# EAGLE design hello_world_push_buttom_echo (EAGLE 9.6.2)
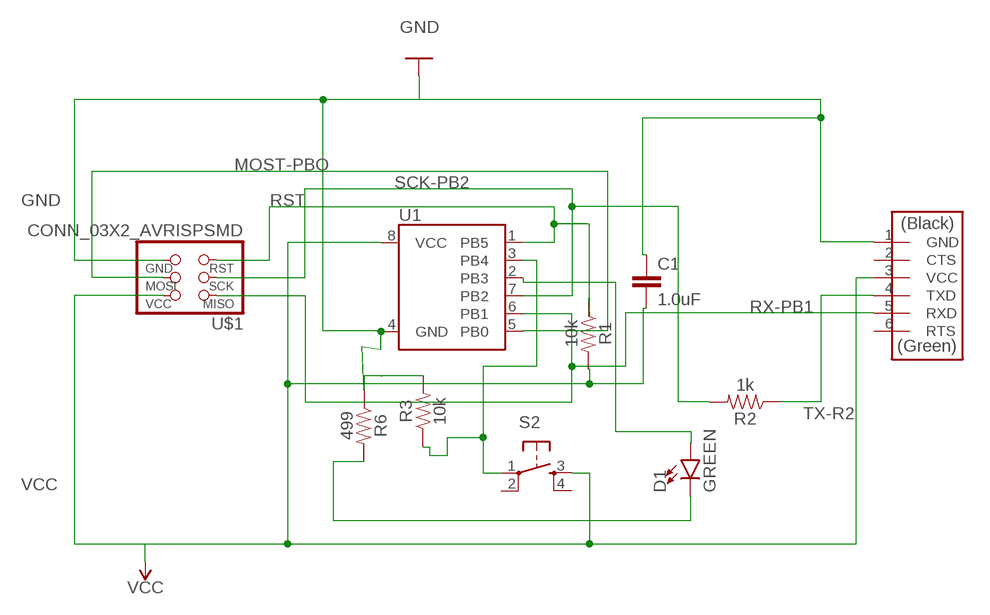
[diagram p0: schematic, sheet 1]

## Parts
C1  1.0uF  1.0UF-1206-50V-10%  [1206]
D1  GREEN  LED-GREEN1206  [LED-1206]
R1  10k  10OHM-1206-1/4W-1%  [1206]
R2  1k  10OHM-1206-1/4W-1%  [1206]
R3  10k  10OHM-1206-1/4W-1%  [1206]
R6  499  10OHM-1206-1/4W-1%  [1206]
S2  6MM_SWITCH6MM_SWITCH  [6MM_SWITCH]
U1  ATTINY85  [ATTINY85]
U$1  CONN_03X2_AVRISPSMD  [2X03SMD]
U$2  CONN_06_FTDI-SMD-HEADER  [1X06SMD]

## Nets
GND: C1.1 R3.2 R6.1 U1.4(GND) U$1.6(GND) U$2.1(GND)
MOST-PBO: U1.5(PB0) U$1.4(MOSI)
N$3: R3.1 S2.1(P) U1.3(PB4)
N$10: D1.A U1.2(PB3)
N$11: D1.C R6.2
RST: R1.1 U1.1(PB5) U$1.5(RST)
RX-PB1: U1.6(PB1) U$1.1(MISO) U$2.5(RXD)
SCK-PB2: R2.2 U1.7(PB2) U$1.3(SCK)
TX-R2: R2.1 U$2.4(TXD)
VCC: C1.2 R1.2 S2.3(S) U1.8(VCC) U$1.2(VCC) U$2.3(VCC)
Unconnected: S2.2(P1) S2.4(S1) U$2.2(CTS) U$2.6(RTS)

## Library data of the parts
C1 = SparkFun-Capacitors:1.0UF: 1µF ceramic capacitors; PROD_ID: CAP-09822
D1 = SparkFun-LED:LED-GREEN: Green SMD LED; PROD_ID: DIO-00862
R1-R3 R6 = SparkFun-Resistors:10OHM: 10Ω resistor; PROD_ID: RES-08705; VALUE: 10
S2 = fab:6MM_SWITCH: OMRON SWITCH
U1 = SparkFun-IC-Microcontroller:ATTINY85; PROD_ID: IC-09092
U$1 = fab:CONN_03X2_AVRISP
U$2 = fab:CONN_06_FTDI-SMD-HEADER

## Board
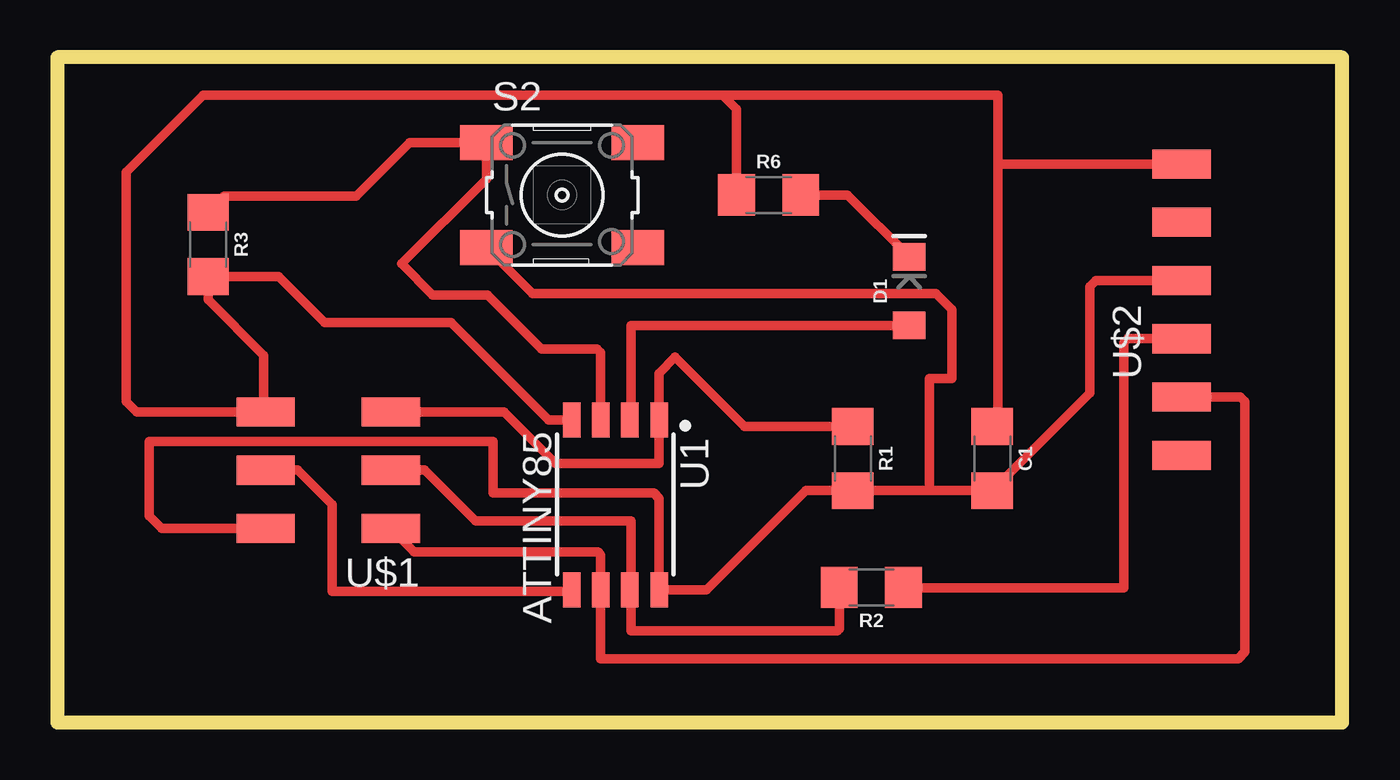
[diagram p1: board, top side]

Size 56 x 29 mm. Coordinates in mm from the lower left corner, seen from the top.
Outline: 0,0 56,0 56,29 0,29 0,0
Copper layers (1*16): Top 0.035mm / dielectric 1.5mm / Bottom 0.035mm
Design rules "default": minimum track width 6mil, minimum drill 0.35mm, track to track 6mil, track to pad 6mil, pad to pad 6mil, via to via 6mil, smd to smd 6mil, copper to edge 40mil, drill to drill 6mil, minimum pad ring 10mil, minimum via ring 8mil, stop-mask expansion 4mil, vias tented up to drill 0mil, thermal gap 10mil

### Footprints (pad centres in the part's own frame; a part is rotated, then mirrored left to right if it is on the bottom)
1206 = smd 1.6 x 1.8: 1 -1.4,0; 2 1.4,0
LED-1206 = smd 1.2 x 1.4: A -1.5,0; C 1.5,0
6MM_SWITCH = smd 2.286 x 1.524: 1 -3.302,2.286; 2 3.302,2.286; 3 -3.302,-2.286; 4 3.302,-2.286
ATTINY85 = smd 1.524 x 0.762: 1 -3.683,1.905; 2 -3.683,0.635; 3 -3.683,-0.635; 4 -3.683,-1.905; 5 3.727,-1.905; 6 3.727,-0.635; 7 3.727,0.635; 8 3.727,1.905
2X03SMD = smd 2.54 x 1.27: 1 -2.54,2.54; 2 2.92,2.54; 3 -2.54,0; 4 2.92,0; 5 -2.54,-2.54; 6 2.92,-2.54
1X06SMD = smd 2.54 x 1.27: 1 0,6.35; 2 0,3.81; 3 0,1.27; 4 0,-1.27; 5 0,-3.81; 6 0,-6.35

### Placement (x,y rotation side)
C1  40.75,11.51 270 top
D1  37.13,18.81 90 top
R1  34.67,11.51 270 top
R2  35.48,5.89 180 top
R3  6.57,20.84 270 top
R6  31,23 0 top
S2  22,23 0 top
U1  24.32,9.51 270 top
U$1  12,11 180 top
U$2  49,18 0 top

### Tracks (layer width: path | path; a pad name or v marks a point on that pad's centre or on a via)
GND
  Top 0.406: 29,27.35 6.35,27.35 3,24 3,14 3.46,13.54 U$1.6 9,13.62 9,16 6.57,18.43 R3.2 9.64,19.44 11.64,17.44 17.17,17.44 21.41,13.19 U1.4 | 29,27.35 41,27.35 41,24.35 | 41,24.35 U$2.1 | C1.1 41,13.16 41,24.35 | R6.1 29.6,26.75 29,27.35
MOST-PBO
  Top 0.406: U$1.4 10.48,11 11.98,9.5 11.98,5.71 22.34,5.71 U1.5
N$3
  Top 0.406: R3.1 7.28,22.95 13.01,22.95 15.35,25.29 S2.1 18.7,23.7 15,20 16.36,18.64 18.75,18.64 21.11,16.28 23.53,16.28 23.68,16.12 U1.3
N$10
  Top 0.406: D1.A 25,17.31 25,13.24 U1.2
N$11
  Top 0.406: D1.C 34.44,23 R6.2
RST
  Top 0.406: U$1.5 19.46,13.54 21.71,11.29 26.23,11.29 U1.1 26.23,15.23 26.93,15.93 29.94,12.91 R1.1
RX-PB1
  Top 0.406: U$1.1 15.56,7.44 23.56,7.44 23.68,7.32 U1.6 23.85,5.61 23.67,5.43 23.67,2.78 51.47,2.78 51.76,3.07 51.76,14 51.57,14.19 U$2.5
SCK-PB2
  Top 0.406: U$1.3 16,11 18.22,8.78 25,8.78 25,5.83 U1.7 25,5.74 25,4 34,4 34.08,4.08 R2.2
TX-R2
  Top 0.406: 48.85,16.73 U$2.4 46.65,16.73 46.49,16.57 46.49,5.86 36.91,5.86 R2.1
VCC
  Top 0.406: U$1.2 4.54,8.46 4,9 4,12.26 19,12.26 19,10 26,10 26.23,9.77 U1.8 28.3,5.78 32.62,10.11 R1.2 38,10.11 | 38,10.11 C1.2 45,14.36 45,19 45.27,19.27 U$2.3 | S2.3 20.7,18.71 38.29,18.71 39,18 39,15 38,15 38,10.11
